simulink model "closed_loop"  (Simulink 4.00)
settings: Solver=ode45  StartTime=0.0  StopTime=10.0  RelTol=1e-3
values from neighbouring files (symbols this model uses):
  d = 1    [EXAMPLE1.M]    (also in EXAMPLE2.M)
  r = 1    [EXAMPLE1.M]    (also in EXAMPLE2.M)
  Td = 5    [EXAMPLE1.M]    (also in EXAMPLE2.M)
  Tr = 1    [EXAMPLE1.M]    (also in EXAMPLE2.M)
libraries: cstblocks x2

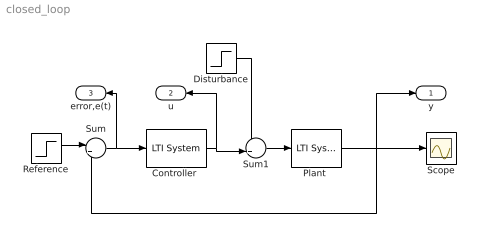
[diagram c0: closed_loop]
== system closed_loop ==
  "Controller " : cstblocks/LTI System  sys=C  IC=[]
  Disturbance : Step  Time=Td  Before=0  After=d  SampleTime=0
  "Plant " : cstblocks/LTI System  sys=Go  IC=[]
  Reference : Step  Time=Tr  Before=0  After=r  SampleTime=0
  Scope : Scope
  Sum : Sum  Inputs=|+-  SaturateOnIntegerOverflow=on
  Sum1 : Sum  Inputs=++|  SaturateOnIntegerOverflow=on
  y : Outport  Port=1
  u : Outport  Orientation=left  Port=2
  error,e(t) : Outport  Orientation=left  Port=3
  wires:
  "Controller "/1 -> Sum1/2, u/1
  Sum1/1 -> "Plant "/1
  "Plant "/1 -> Scope/1, Sum/2, y/1
  Sum/1 -> "Controller "/1, error,e(t)/1
  Reference/1 -> Sum/1
  Disturbance/1 -> Sum1/1
